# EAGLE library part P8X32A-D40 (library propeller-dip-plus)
Parallax Propeller P8X32A-D40 Microcontroller DIP40
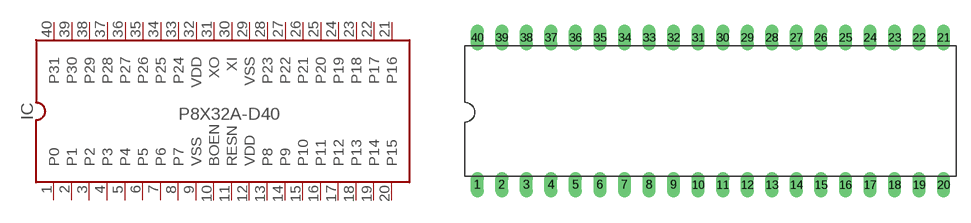
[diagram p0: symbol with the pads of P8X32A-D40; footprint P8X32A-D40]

Designator prefix IC

## P8X32A-D40DIP-40  [P8X32A-D40]
1  P0
2  P1
3  P2
4  P3
5  P4
6  P5
7  P6
8  P7
9  VSS  pwr
10  BOEN  in
11  RESN
12  VDD  pwr
13  P8
14  P9
15  P10
16  P11
17  P12
18  P13
19  P14
20  P15
21  P16
22  P17
23  P18
24  P19
25  P20
26  P21
27  P22
28  P23
29  VSS  pwr
30  XI  in
31  XO  out
32  VDD  pwr
33  P24
34  P25
35  P26
36  P27
37  P28
38  P29
39  P30
40  P31

## Footprint P8X32A-D40 (pad centres in mm)
Parallax Propeller P8X32A-D40 Microcontroller DIP40
drill 0.813 long: 1 -22.86,-8.89; 2 -20.32,-8.89; 3 -17.78,-8.89; 4 -15.24,-8.89; 5 -12.7,-8.89; 6 -10.16,-8.89; 7 -7.62,-8.89; 8 -5.08,-8.89; 9 -2.54,-8.89; 10 0,-8.89; 11 2.54,-8.89; 12 5.08,-8.89; 13 7.62,-8.89; 14 10.16,-8.89; 15 12.7,-8.89; 16 15.24,-8.89; 17 17.78,-8.89; 18 20.32,-8.89; 19 22.86,-8.89; 20 25.4,-8.89; 21 25.4,6.35; 22 22.86,6.35; 23 20.32,6.35; 24 17.78,6.35; 25 15.24,6.35; 26 12.7,6.35; 27 10.16,6.35; 28 7.62,6.35; 29 5.08,6.35; 30 2.54,6.35; 31 0,6.35; 32 -2.54,6.35; 33 -5.08,6.35; 34 -7.62,6.35; 35 -10.16,6.35; 36 -12.7,6.35; 37 -15.24,6.35; 38 -17.78,6.35; 39 -20.32,6.35; 40 -22.86,6.35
